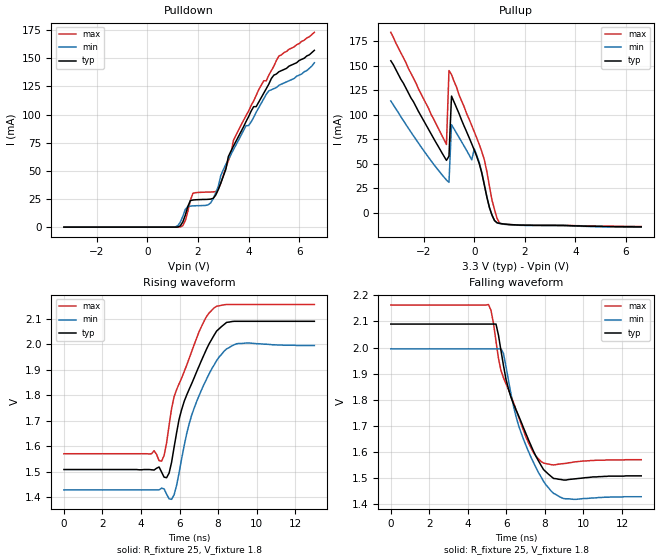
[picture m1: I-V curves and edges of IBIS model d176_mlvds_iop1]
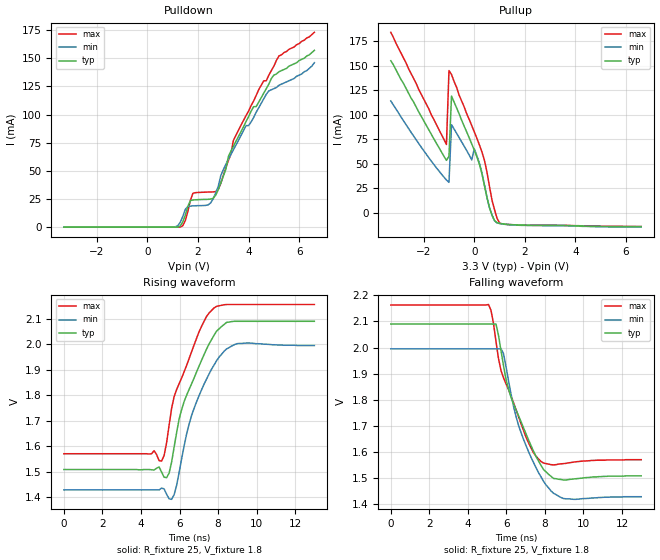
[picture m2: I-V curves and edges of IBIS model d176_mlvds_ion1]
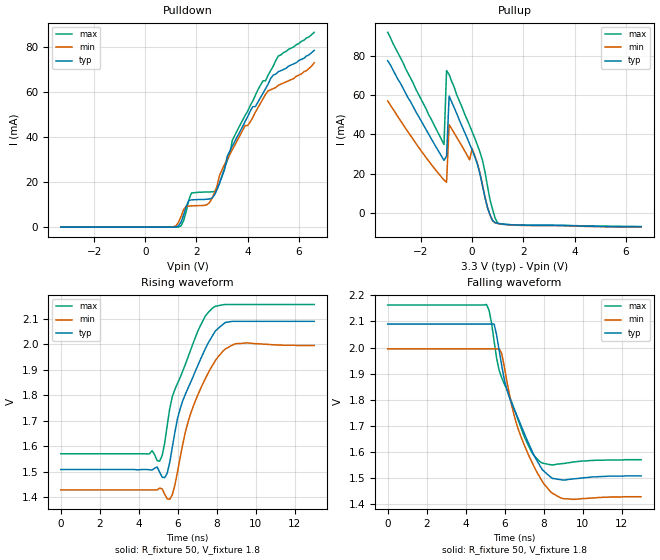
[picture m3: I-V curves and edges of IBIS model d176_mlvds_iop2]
|   National Semiconductor Corporation
|   IBIS Model
|   of
|   DS91D176
|   3.3V M-LVDS Multipoint Transceivers
[IBIS Ver]   3.2
[Comment Char]   |_char
[File name]   ds91d176tma.ibs
[File Rev]   1.1
[Date]   04/19/06
[Source]
Spectre simulations
[Notes]
Created by Ivan Duzevik
Version 1.1   Updated mlvds_io models - dglisic
[Disclaimer]
(C) Copyright National Semiconductor Corporation 2005
   All rights reserved
   National Semiconductor Corporation hereby grants
the user of this IBIS model a non-exclusive, nontransferable
license to use this IBIS model under the following terms.
Before using this IBIS model, the user should read this
license.  If the user does not accept these terms,  the
IBIS model should be returned to National within 30 days.
   The user is granted this license only to use the
IBIS model and is not granted rights to sell, load, rent,
lease or license the IBIS model in whole or in part, or in
modified form to anyone other than user. User may modify
the IBIS model to suit its specific applications but rights
to derivative works and such modifications shall belong to
National.
   This IBIS model is provided on an "AS IS" basis and
National makes absolutely no warranty with respect to the
information contained herein.NATIONAL DISCLAIMS AND CUSTOMER
WAIVES ALL WARRANTIES, EXPRESS OR IMPLIED, INCLUDING
WARRANTIES OF MERCHANTABILITY OR FITNESS FOR A PARTICULAR
PURPOSE. The entire risk as to quality and performance is
with the Customer. ACCORDINGLY, IN NO EVENT SHALL THE
COMPANY BE LIABLE FOR ANY DAMAGES, WHETHER IN CONTRACT OR
TORT,INCLUDING ANY LOST PROFITS OR OTHER INCIDENTAL,
CONSEQUENTIAL, EXEMPLARY, OR PUNITIVE DAMAGES ARISING OUT
OF THE USE OR APPLICATION OF THE IBIS model provided in
this package.Further, National reserves the right to make
changes without notice to any product herein to improve
reliability, function, or design. National does not convey
any license under patent rights or any other intellectual
property rights, including those of third parties.
   National is not obligated to provide maintenance or support
for the licensed IBIS model.
Contact National at ATTN:INTERFACE/IBIS MODELS.
5 Foden Road, M/S 01-50, South Porltand, ME 04106
(207) 541-8467
[Copyright]
(c) Copyright 2005 National Semiconductor Corp.
[Component]   DS91D176
Si_location Pin
Timing_location Pin
[Manufacturer]   National Semiconductor Corp.
[Package]
|   TYP   MIN   MAX
R_pkg   50.0m   50.0m   50.0m
L_pkg   1.164nH   1.040nH   1.330nH
C_pkg   0.207pF   0.178pF   0.245pF
[Pin]   signal_name   model_name   R_pin   L_pin   C_pin
1   R   d176_cmos_out   50.0m   1.33n   0.245p
2   REb   d176_cmos_in   50.0m   1.04n   0.178p
3   DE   d176_cmos_in   50.0m   1.04n   0.178p
4   D   d176_cmos_in   50.0m   1.33n   0.178p
5   GND   POWER   50.0m   1.33n   0.245p
6   A   d176_mlvds_iop   50.0m   1.04n   0.178p
7   B   d176_mlvds_ion   50.0m   1.04n   0.178p
8   VDD   POWER   50.0m   1.33n   0.245p
[Diff Pin] inv_pin   vdiff   tdelay_typ   tdelay_min   tdelay_max
| The '+' pin is Diff_pin and the '-' pin is the inv_pin
| Receiver Vth = +/-50mV
6   7   0.05   0   0   0
[Model Selector]   d176_mlvds_iop
d176_mlvds_iop1   Use this model for 50-ohm loads
d176_mlvds_iop2   Use this model for 100-ohm loads
[Model Selector]   d176_mlvds_ion
d176_mlvds_ion1   Use this model for 50-ohm loads
d176_mlvds_ion2   Use this model for 100-ohm loads
| Models and submodels in the file (6): d176_mlvds_iop1 (I/O), d176_mlvds_ion1 (I/O), d176_mlvds_iop2 (I/O), d176_mlvds_ion2 (I/O), d176_cmos_out (Output), d176_cmos_in (Input)
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[Model]   d176_mlvds_iop1
Model_type I/O
Polarity Non-Inverting
Vinh=0.05
Vinl=-0.05
Vref=1.8
Vmeas=1.8
Rref=25
Cref=0p
|   Typ   Min   Max
C_comp   9.5pF   9.5pF   9.5pF
[Model Spec]
S_overshoot_high   3.8   3.8   3.8
S_overshoot_low   -1.4   -1.4   -1.4
[Temperature Range]   25   85   -40
[Voltage Range]   3.3   3.0   3.6
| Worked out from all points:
|   slope of the pullup table from 0 to 0.495 V, typ, clamps not added: 10.4 ohm
|   rising waveform, R_fixture 25, V_fixture 1.8: 20-80 % time 1.58ns typ, 1.44ns min, 1.49ns max; typ from 1.51 V to 2.09 V
|   falling waveform, R_fixture 25, V_fixture 1.8: 20-80 % time 1.52ns typ, 1.44ns min, 1.44ns max; typ from 2.09 V to 1.51 V
[GND Clamp]
|V(groundclamp)   I(typ)   I(min)   I(max)
-3.3V     0A         0A         0A
3.3V      0A         0A         0A
[POWER Clamp]
|V(powerclamp)   I(typ)   I(min)   I(max)
-3.3V     0A         0A         0A
0V        0A         0A         0A
[Pullup]
|Vtable   I(typ)   I(min)   I(max)
-3.3V     155mA      114mA      184mA
-2.1V     98.5mA     67mA       121mA
-1.1V     53.4mA     33.4mA     69.6mA
-1V       57.7mA     31mA       145mA
-900mV    119mA      89.8mA     141mA
-100mV    70.2mA     53.9mA     88.9mA
0V        63.9mA     65.2mA     82.5mA
200mV     49.8mA     50.8mA     69.4mA
400mV     28mA       28.6mA     53.7mA
700mV     -2.35mA    -2.4mA     12.9mA
1V        -10.8mA    -11mA      -10.5mA
6.6V      -14.4mA    -14.7mA    -14mA
[Pulldown]
|V(pulldown)   I(typ)   I(min)   I(max)
-3.3V     -27.9pA    -146pA     -28.2pA
1.1V      12.8uA     221uA      140nA
1.4V      4.61mA     9.58mA     1.28mA
1.7V      23.6mA     18.7mA     23.9mA
1.8V      24.1mA     18.9mA     30.1mA
2.5V      24.9mA     21.5mA     31.2mA
2.8V      33.2mA     36.1mA     33.6mA
3.3V      67.4mA     64.4mA     64.7mA
3.4V      71.9mA     68.7mA     77mA
4.7V      123mA      118mA      130mA
5.2V      138mA      126mA      152mA
6.6V      157mA      146mA      173mA
[Rising Waveform]
R_fixture=25
V_fixture=1.8
V_fixture_min=1.72
V_fixture_max=1.86
0s        1.508V     1.428V     1.57V
4.68ns    1.506V     1.428V     1.582V
5.07ns    1.498V     1.435V     1.541V
5.33ns    1.476V     1.411V     1.613V
5.59ns    1.537V     1.391V     1.748V
6.24ns    1.775V     1.601V     1.892V
6.63ns    1.845V     1.721V     1.971V
7.41ns    1.982V     1.864V     2.11V
8.32ns    2.078V     1.973V     2.155V
13ns      2.09V      1.995V     2.156V
[Falling Waveform]
R_fixture=25
V_fixture=1.8
V_fixture_min=1.72
V_fixture_max=1.86
0s        2.09V      1.995V     2.163V
5.07ns    2.09V      1.995V     2.165V
5.46ns    2.09V      1.995V     2.024V
5.72ns    1.988V     1.995V     1.912V
6.11ns    1.841V     1.873V     1.839V
6.76ns    1.716V     1.674V     1.708V
7.41ns    1.602V     1.559V     1.596V
8.32ns    1.506V     1.45V      1.551V
9.49ns    1.496V     1.418V     1.561V
13ns      1.508V     1.428V     1.57V
[Ramp]
|   typ   min   max
dV/dt_r   340m/1054p   340m/1350p   340m/806p
dV/dt_f   340m/1054p   340m/1350p   340m/806p
R_load=50
|[End   ds91d176_mlvds_io1
[Model]   d176_mlvds_ion1
Model_type I/O
Polarity Inverting
Vinh=0.05
Vinl=-0.05
Vref=1.8
Vmeas=1.8
Rref=25
Cref=0p
|   Typ   Min   Max
C_comp   9.5pF   9.5pF   9.5pF
[Model Spec]
S_overshoot_high   3.8   3.8   3.8
S_overshoot_low   -1.4   -1.4   -1.4
[Temperature Range]   25   85   -40
[Voltage Range]   3.3   3.0   3.6
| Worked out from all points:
|   slope of the pullup table from 0 to 0.495 V, typ, clamps not added: 10.4 ohm
|   rising waveform, R_fixture 25, V_fixture 1.8: 20-80 % time 1.58ns typ, 1.44ns min, 1.49ns max; typ from 1.51 V to 2.09 V
|   falling waveform, R_fixture 25, V_fixture 1.8: 20-80 % time 1.52ns typ, 1.44ns min, 1.44ns max; typ from 2.09 V to 1.51 V
[GND Clamp]
|V(groundclamp)   I(typ)   I(min)   I(max)
-3.3V     0A         0A         0A
3.3V      0A         0A         0A
[POWER Clamp]
|V(powerclamp)   I(typ)   I(min)   I(max)
-3.3V     0A         0A         0A
0V        0A         0A         0A
[Pullup]
|Vtable   I(typ)   I(min)   I(max)
-3.3V     155mA      114mA      184mA
-2.1V     98.5mA     67mA       121mA
-1.1V     53.4mA     33.4mA     69.6mA
-1V       57.7mA     31mA       145mA
-900mV    119mA      89.8mA     141mA
-100mV    70.2mA     53.9mA     88.9mA
0V        63.9mA     65.2mA     82.5mA
200mV     49.8mA     50.8mA     69.4mA
400mV     28mA       28.6mA     53.7mA
700mV     -2.35mA    -2.4mA     12.9mA
1V        -10.8mA    -11mA      -10.5mA
6.6V      -14.4mA    -14.7mA    -14mA
[Pulldown]
|V(pulldown)   I(typ)   I(min)   I(max)
-3.3V     -27.9pA    -146pA     -28.2pA
1.1V      12.8uA     221uA      140nA
1.4V      4.61mA     9.58mA     1.28mA
1.7V      23.6mA     18.7mA     23.9mA
1.8V      24.1mA     18.9mA     30.1mA
2.5V      24.9mA     21.5mA     31.2mA
2.8V      33.2mA     36.1mA     33.6mA
3.3V      67.4mA     64.4mA     64.7mA
3.4V      71.9mA     68.7mA     77mA
4.7V      123mA      118mA      130mA
5.2V      138mA      126mA      152mA
6.6V      157mA      146mA      173mA
[Rising Waveform]
R_fixture=25
V_fixture=1.8
V_fixture_min=1.72
V_fixture_max=1.86
0s        1.508V     1.428V     1.57V
4.68ns    1.506V     1.428V     1.582V
5.07ns    1.498V     1.435V     1.541V
5.33ns    1.476V     1.411V     1.613V
5.59ns    1.537V     1.391V     1.748V
6.24ns    1.775V     1.601V     1.892V
6.63ns    1.845V     1.721V     1.971V
7.41ns    1.982V     1.864V     2.11V
8.32ns    2.078V     1.973V     2.155V
13ns      2.09V      1.995V     2.156V
[Falling Waveform]
R_fixture=25
V_fixture=1.8
V_fixture_min=1.72
V_fixture_max=1.86
0s        2.09V      1.995V     2.163V
5.07ns    2.09V      1.995V     2.165V
5.46ns    2.09V      1.995V     2.024V
5.72ns    1.988V     1.995V     1.912V
6.11ns    1.841V     1.873V     1.839V
6.76ns    1.716V     1.674V     1.708V
7.41ns    1.602V     1.559V     1.596V
8.32ns    1.506V     1.45V      1.551V
9.49ns    1.496V     1.418V     1.561V
13ns      1.508V     1.428V     1.57V
[Ramp]
|   typ   min   max
dV/dt_r   340m/1054p   340m/1350p   340m/806p
dV/dt_f   340m/1054p   340m/1350p   340m/806p
R_load=50
|[End   ds91d176_mlvds_io1
[Model]   d176_mlvds_iop2
Model_type I/O
Polarity Non-Inverting
Vinh=0.05
Vinl=-0.05
Vref=1.8
Vmeas=1.8
Rref=50
Cref=0p
|   Typ   Min   Max
C_comp   9.5pF   9.5pF   9.5pF
[Model Spec]
S_overshoot_high   3.8   3.8   3.8
S_overshoot_low   -1.4   -1.4   -1.4
[Temperature Range]   25   85   -40
[Voltage Range]   3.3   3.0   3.6
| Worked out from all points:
|   slope of the pullup table from 0 to 0.495 V, typ, clamps not added: 20.8 ohm
|   rising waveform, R_fixture 50, V_fixture 1.8: 20-80 % time 1.58ns typ, 1.44ns min, 1.49ns max; typ from 1.51 V to 2.09 V
|   falling waveform, R_fixture 50, V_fixture 1.8: 20-80 % time 1.52ns typ, 1.44ns min, 1.44ns max; typ from 2.09 V to 1.51 V
[GND Clamp]
|V(groundclamp)   I(typ)   I(min)   I(max)
-3.3V     0A         0A         0A
3.3V      0A         0A         0A
[POWER Clamp]
|V(powerclamp)   I(typ)   I(min)   I(max)
-3.3V     0A         0A         0A
0V        0A         0A         0A
[Pullup]
|Vtable   I(typ)   I(min)   I(max)
-3.3V     77.5mA     57mA       92mA
-1.1V     26.7mA     16.7mA     34.8mA
-1V       28.9mA     15.5mA     72.5mA
-900mV    59.5mA     44.9mA     70.5mA
-100mV    35.1mA     27mA       44.5mA
0V        32mA       32.6mA     41.3mA
200mV     24.9mA     25.4mA     34.7mA
400mV     14mA       14.3mA     26.9mA
700mV     -1.18mA    -1.2mA     6.45mA
900mV     -5.1mA     -5.2mA     -2.87mA
1V        -5.4mA     -5.5mA     -5.25mA
6.6V      -7.2mA     -7.35mA    -7mA
[Pulldown]
|V(pulldown)   I(typ)   I(min)   I(max)
-3.3V     -14pA      -73pA      -14.1pA
1.1V      6.4uA      111uA      70nA
1.4V      2.31mA     4.79mA     640uA
1.7V      11.8mA     9.35mA     12mA
1.8V      12.1mA     9.45mA     15.1mA
2.4V      12.4mA     9.9mA      15.6mA
2.8V      16.6mA     18.1mA     16.8mA
3.3V      33.7mA     32.2mA     32.4mA
3.4V      36mA       34.4mA     38.5mA
4.7V      61.5mA     59mA       65mA
5.2V      69mA       63mA       76mA
6.6V      78.5mA     73mA       86.5mA
[Rising Waveform]
R_fixture=50
V_fixture=1.8
V_fixture_min=1.72
V_fixture_max=1.86
0s        1.508V     1.428V     1.57V
4.68ns    1.506V     1.428V     1.582V
5.07ns    1.498V     1.435V     1.541V
5.33ns    1.476V     1.411V     1.613V
5.59ns    1.537V     1.391V     1.748V
6.24ns    1.775V     1.601V     1.892V
6.63ns    1.845V     1.721V     1.971V
7.41ns    1.982V     1.864V     2.11V
8.32ns    2.078V     1.973V     2.155V
13ns      2.09V      1.995V     2.156V
[Falling Waveform]
R_fixture=50
V_fixture=1.8
V_fixture_min=1.72
V_fixture_max=1.86
0s        2.09V      1.995V     2.163V
5.07ns    2.09V      1.995V     2.165V
5.46ns    2.09V      1.995V     2.024V
5.72ns    1.988V     1.995V     1.912V
6.11ns    1.841V     1.873V     1.839V
6.76ns    1.716V     1.674V     1.708V
7.41ns    1.602V     1.559V     1.596V
8.32ns    1.506V     1.45V      1.551V
9.49ns    1.496V     1.418V     1.561V
13ns      1.508V     1.428V     1.57V
[Ramp]
|   typ   min   max
dV/dt_r   340m/1054p   340m/1350p   340m/806p
dV/dt_f   340m/1054p   340m/1350p   340m/806p
R_load=50
|[End   ds91d176_mlvds_io2
